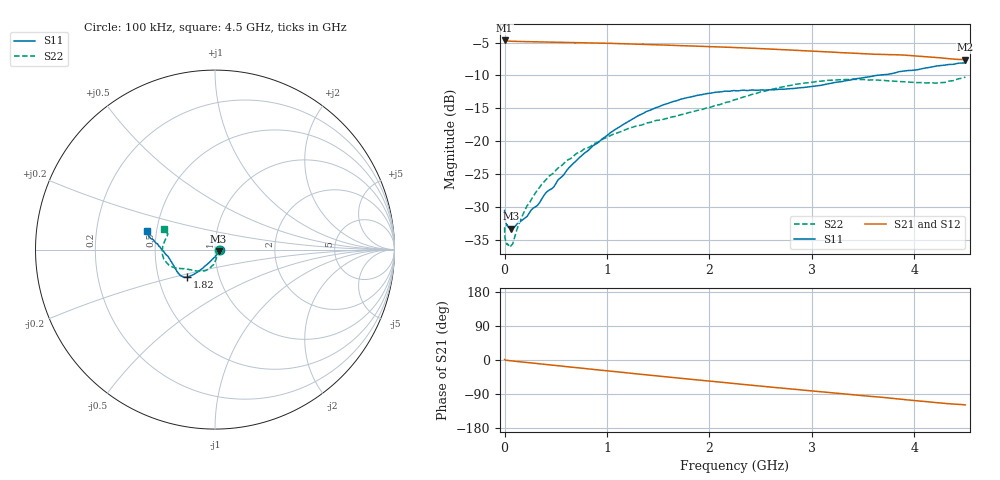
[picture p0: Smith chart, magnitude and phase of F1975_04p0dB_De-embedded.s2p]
! Integrated Device Technology
! Corporate Headquarters
! 6024 Silver Creek Valley Road
! San Jose, CA 95138  USA
! Phone:  1-408-284-8200
! Toll Free:  1-800-223-1366
! Webpage:  http://www.idt.com/
! Timing and RF Division
! 515 Groton Road, Suite 102
! Westford, MA 01886-6024
! Device:  F1975
! Description: 6-bit, 75 ohm, 0.5 dB Digital Step Attenuator
! Frequency:  5.0 MHz -  3.00 GHz
! Package:  4x4 mm QFN Plastic Package: 20 pin
! Ports:  2 RF, 11 DC
!  Pin  1  = D5 (16 dB)
!  Pin  2  = RF1  =  Port 1
!  Pin  3  = Serial Data In (DATA)
!  Pin  4  = Serial Clock (CLK)
!  Pin  5  = Serial Latch Enable (LE)
!  Pin  6  = VDD
!  Pin  7  = NC
!  Pin  8  = NC
!  Pin  9  = NC
!  Pin 10  = GND
!  Pin 11  = GND
!  Pin 12  = NC
!  Pin 13  = VMODE
!  Pin 14  = RF2  =  Port 2
!  Pin 15  = D4 (8 dB)
!  Pin 16  = D3 (4 dB)
!  Pin 17  = D2 (2 dB)
!  Pin 18  = NC
!  Pin 19  = D1 (1 dB)
!  Pin 20  = D0 (0.5 dB)
! State:  8
! Atten State:  4.0 dB
! Voltage:  +3.30 Volts
! Current:  0.595 mA
! Data:  The device was measured on a F1975 evaluation board which has
!  individual transmission lines to the RF pins.  Data was collected
!  using a calibrated network analyzer.  The evaluation board was
!  de-embedded using Automatic Fixture Removal (AFR).
!  The reference plane is the edge of the package pin.
! Misc:
!  Action Tracker AT0415
! Date Measured:  2018-02-08
! Date:  2018-03-26  MJV
! Note:
!  Integrated Device Technology supplies this data as a sample of measured
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# GHz S dB R 75
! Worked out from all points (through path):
!   291 points, 100 kHz to 4.5 GHz, reference 75 ohm
!   highest |S21| = -4.69 dB at 100 kHz (marker M1); lowest = -7.6 dB at 4.5 GHz (marker M2)
!   group delay of S21, straight-line fit = 74.2 ps
!   lowest |S11| = -33.3 dB at 60 MHz (marker M3), VSWR 1.04, Z = 78 - j1.43 ohm
!   |S11| at or under -10 dB: start of sweep to 3.633 GHz
!   |S22| runs from -35.9 to -10.2 dB; largest |S21 - S12| = 0.00022
!   S11 on the Smith chart (normalised r, x): 100 kHz: 1.06, -0.00; 1.82 GHz: 0.70, -0.23; 4.5 GHz: 0.44, +0.11
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0.0001  -30.51 -0.4  -4.69 1.2  -4.69 1.2  -33.05 0.4
0.0007  -31.33 -2.5  -4.72 1.0  -4.72 1.0  -33.95 -3.0
0.002  -31.72 -3.0  -4.73 0.8  -4.73 0.8  -34.43 -3.1
0.015  -32.41 -9.4  -4.77 -0.7  -4.77 -0.7  -35.37 -13.5
0.06  -33.29 -25.1  -4.81 -2.1  -4.81 -2.0  -35.91 -35.3
0.08  -33.18 -32.6  -4.82 -2.6  -4.82 -2.6  -35.55 -46.7
0.12  -32.57 -42.6  -4.84 -3.8  -4.84 -3.8  -33.40 -59.2
0.22  -31.41 -63.2  -4.87 -6.7  -4.87 -6.7  -29.77 -70.7
0.32  -29.76 -78.3  -4.90 -9.5  -4.90 -9.5  -27.39 -78.7
0.4  -27.89 -88.8  -4.92 -11.7  -4.92 -11.7  -25.91 -82.0
0.48  -26.94 -96.6  -4.94 -14.0  -4.94 -14.0  -24.80 -85.9
0.52  -25.92 -100.8  -4.96 -15.1  -4.96 -15.1  -24.10 -87.9
0.76  -22.07 -113.8  -5.03 -21.8  -5.03 -21.8  -21.39 -96.9
1.08  -18.21 -123.3  -5.15 -30.8  -5.14 -30.8  -18.82 -108.0
1.52  -14.67 -130.9  -5.36 -42.8  -5.36 -42.8  -16.78 -123.8
1.82  -13.26 -135.2  -5.53 -50.9  -5.53 -50.9  -15.57 -135.3
2.26  -12.32 -145.1  -5.77 -62.5  -5.76 -62.5  -13.65 -149.0
2.68  -12.10 -159.1  -6.05 -73.6  -6.05 -73.6  -11.84 -157.7
3.02  -11.66 -170.3  -6.32 -82.3  -6.32 -82.3  -10.99 -166.0
3.76  -9.79 174.2  -6.84 -100.3  -6.83 -100.3  -10.83 173.0
4.22  -8.57 169.1  -7.26 -112.6  -7.26 -112.6  -11.16 161.8
4.5  -8.11 164.4  -7.60 -118.4  -7.59 -118.4  -10.24 157.8
